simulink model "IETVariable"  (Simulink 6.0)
settings: Solver=ode45  StartTime=0.0  StopTime=10  RelTol=1e-3
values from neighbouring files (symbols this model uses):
  b = S/Sm    (= 0.1)    [Constantes.m]    (also in ConstantesBck.m)
  beta = 0.95    [Constantes.m]    (also in ConstantesBck.m; ResCourV1.m = 1; ResCrV1.m = 1; ResEnerV1.m = 1)
  C = 1    [Constantes.m]    (also in ConstantesBck.m)
  Cdl = 603E-9    (= 6.03e-07)    [Constantes.m]    (also in ConstantesBck.m; ResCourV1.m = 7.313e-07; ResCrV1.m = 7.313e-07; ResEnerV1.m = 7.313e-07)
  Cmem = 1E-6*Sm*(1-b)    (= 2.826e-08)    [Constantes.m]    (also in ConstantesBck.m = 3.14e-11; ImpedanceZtissus.m = 4e-08; Ztissus.m = 4e-08; CalculCharge.m = 1)
  Fact = 10^2    (= 100)    [Constantes.m]    (also in ConstantesBck.m)
  gk = 36    [Constantes.m]    (also in ConstantesBck.m; sim_hh.m)
  gl = 0.3    [Constantes.m]    (also in ConstantesBck.m; sim_hh.m)
  gna = 120    [Constantes.m]    (also in ConstantesBck.m; sim_hh.m)
  h0 = 0.5961    [Constantes.m]    (also in ConstantesBck.m)
  m0 = 0.0529    [Constantes.m]    (also in ConstantesBck.m)
  mK = 0    [Constantes.m]    (also in ConstantesBck.m)
  mL = 0    [Constantes.m]    (also in ConstantesBck.m)
  mNa = 0    [Constantes.m]    (also in ConstantesBck.m)
  n0 = 0.3177    [Constantes.m]    (also in ConstantesBck.m)
  rapportIE = 10    [Constantes.m]
  Rcan = 6.398E3*Sm*(1-b)    (= 180.80748)    [Constantes.m]    (also in ConstantesBck.m = 0.03454; ImpedanceZtissus.m = 44; Ztissus.m = 44)
  Rct = 185.6E3    (= 185600)    [Constantes.m]    (also in ConstantesBck.m; ResCourV1.m = 605200; ResCrV1.m = 605200; ResEnerV1.m = 605200)
  Rext = 2.9E3    (= 2900)    [Constantes.m]    (also in ConstantesBck.m)
  Rint = 2.9E2    (= 290)    [Constantes.m]    (also in ConstantesBck.m = 400)
  sigma = 66466    [Constantes.m]    (also in ConstantesBck.m; ResCourV1.m = 68000; ResCrV1.m = 68000; ResEnerV1.m = 68000)
  Sm = 3.14e-2    (= 0.0314)    [Constantes.m]    (also in ConstantesBck.m = 0.000314)
  Vk = -82    [Constantes.m]    (also in ConstantesBck.m)
  Vl = -59    [Constantes.m]    (also in ConstantesBck.m)
  Vna = 45    [Constantes.m]    (also in ConstantesBck.m)
  Vr = -70    [Constantes.m]    (also in ConstantesBck.m)
undefined symbols (not defined in the file or in its folder): ln
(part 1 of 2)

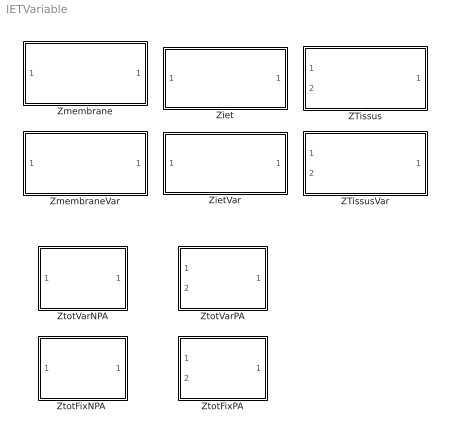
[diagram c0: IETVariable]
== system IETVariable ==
  ZTissus : Subsystem
  ZTissusVar : Subsystem
  Ziet : Subsystem
  ZietVar : Subsystem
  Zmembrane : Subsystem
  ZmembraneVar : Subsystem
  "ZtotFixNPA " : Subsystem
  ZtotFixPA : Subsystem
  ZtotVarNPA : Subsystem
  ZtotVarPA : Subsystem

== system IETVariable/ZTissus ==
  IStim : Inport  Orientation=left  Port=1  LatchInput=off
  Vref : Inport  Port=2  LatchInput=off
  Constant : Constant
  Contrôleur : Stateflow chart  Orientation=left
  Divide : Product  Inputs=*/  OutScaling=2^-10
  Divide1 : Product  Inputs=*/  OutScaling=2^-10
  Divide2 : Product  Inputs=*/  OutScaling=2^-10
  Gain2 : Gain  Gain=Rext
  Sum1 : Sum  Inputs=|++
  ZTissusInt : Subsystem
  Vout : Outport  Orientation=left
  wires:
  Constant/1 -> Divide/1, Divide1/1, Divide2/1
  ZTissusInt/1(Vout) -> Divide/2
  Gain2/1 -> Divide1/2
  Divide/1 -> Sum1/1
  Divide1/1 -> Sum1/2
  Sum1/1 -> Divide2/2
  Vref/1 -> ZTissusInt/2(VRefIn)
  Divide2/1 -> Contrôleur/2(calc)
  Contrôleur/2(temp) -> ZTissusInt/1(InStim), Gain2/1
  IStim/1 -> Contrôleur/1(u)
  Contrôleur/1(y) -> Vout/1

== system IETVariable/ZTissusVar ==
  IStim : Inport  Orientation=left  Port=1  LatchInput=off
  Vref : Inport  Port=2  LatchInput=off
  Constant : Constant
  Contrôleur : Stateflow chart  Orientation=left
  Divide : Product  Inputs=*/  OutScaling=2^-10
  Divide1 : Product  Inputs=*/  OutScaling=2^-10
  Divide2 : Product  Inputs=*/  OutScaling=2^-10
  Rext1 : Fcn  Expr=u*(1.6342*((abs(u)*1E6)^0.1267))*1E3
  Sum1 : Sum  Inputs=|++
  ZTissusInt1 : Subsystem
  Vout : Outport  Orientation=left
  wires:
  Constant/1 -> Divide/1, Divide1/1, Divide2/1
  ZTissusInt1/1(Vout) -> Divide/2
  Rext1/1 -> Divide1/2
  Divide/1 -> Sum1/1
  Divide1/1 -> Sum1/2
  Sum1/1 -> Divide2/2
  Vref/1 -> ZTissusInt1/2(VRefIn)
  Divide2/1 -> Contrôleur/2(calc)
  Contrôleur/2(temp) -> Rext1/1, ZTissusInt1/1(InStim)
  IStim/1 -> Contrôleur/1(u)
  Contrôleur/1(y) -> Vout/1

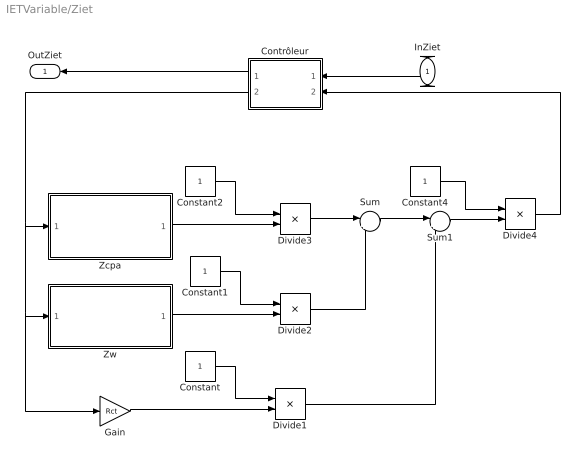
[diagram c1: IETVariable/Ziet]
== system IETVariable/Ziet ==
  InZiet : Inport  Orientation=left  Port=1  LatchInput=off
  Constant{,1..2,4} (4 alike) : Constant
  Contrôleur : Stateflow chart  Orientation=left
  Divide{1..4} (4 alike) : Product  Inputs=*/  OutScaling=2^-10
  Gain : Gain  Gain=Rct
  Sum : Sum  Inputs=|++
  Sum1 : Sum  Inputs=|++
  Zcpa : Subsystem
  Zw : Subsystem
  OutZiet : Outport  Orientation=left
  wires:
  Constant/1 -> Divide1/1
  Constant1/1 -> Divide2/1
  Constant2/1 -> Divide3/1
  Zcpa/1(OutZcpa) -> Divide3/2
  Zw/1(OutZw) -> Divide2/2
  Divide3/1 -> Sum/1
  Constant4/1 -> Divide4/1
  Divide2/1 -> Sum/2
  Sum/1 -> Sum1/1
  Divide1/1 -> Sum1/2
  Sum1/1 -> Divide4/2
  Divide4/1 -> Contrôleur/2(calc)
  Gain/1 -> Divide1/2
  InZiet/1 -> Contrôleur/1(u)
  Contrôleur/1(y) -> OutZiet/1
  Contrôleur/2(temp) -> Zcpa/1(InZcpa), Zw/1(InZw), Gain/1

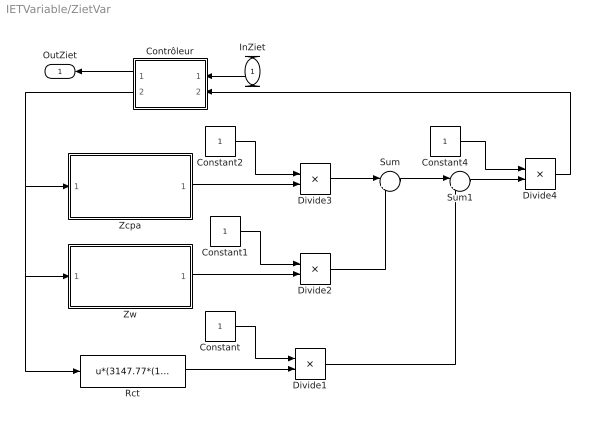
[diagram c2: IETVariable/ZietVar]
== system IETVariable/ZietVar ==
  InZiet : Inport  Orientation=left  Port=1  LatchInput=off
  Constant{,1..2,4} (4 alike) : Constant
  Contrôleur : Stateflow chart  Orientation=left
  Divide{1..4} (4 alike) : Product  Inputs=*/  OutScaling=2^-10
  Rct : Fcn  Expr=u*(3147.77*(1/((1E6*abs(u))^0.7199)))*1000
  Sum : Sum  Inputs=|++
  Sum1 : Sum  Inputs=|++
  Zcpa : Subsystem
  Zw : Subsystem
  OutZiet : Outport  Orientation=left
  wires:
  Constant/1 -> Divide1/1
  Constant1/1 -> Divide2/1
  Constant2/1 -> Divide3/1
  Zcpa/1(OutZcpa) -> Divide3/2
  Zw/1(OutZw) -> Divide2/2
  Rct/1 -> Divide1/2
  Divide3/1 -> Sum/1
  Constant4/1 -> Divide4/1
  Divide2/1 -> Sum/2
  Sum/1 -> Sum1/1
  Divide1/1 -> Sum1/2
  Sum1/1 -> Divide4/2
  Contrôleur/2(temp) -> Rct/1, Zw/1(InZw), Zcpa/1(InZcpa)
  InZiet/1 -> Contrôleur/1(u)
  Contrôleur/1(y) -> OutZiet/1
  Divide4/1 -> Contrôleur/2(calc)

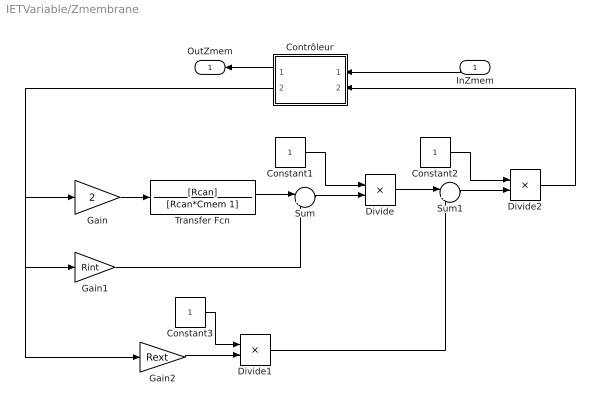
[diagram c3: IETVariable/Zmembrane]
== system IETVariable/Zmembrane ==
  InZmem : Inport  Orientation=left  Port=1  LatchInput=off
  Constant1 : Constant
  Constant2 : Constant
  Constant3 : Constant
  Contrôleur : Stateflow chart  Orientation=left
  Divide : Product  Inputs=*/  OutScaling=2^-10
  Divide1 : Product  Inputs=*/  OutScaling=2^-10
  Divide2 : Product  Inputs=*/  OutScaling=2^-10
  Gain : Gain  Gain=2
  Gain1 : Gain  Gain=Rint
  Gain2 : Gain  Gain=Rext
  Sum : Sum  Inputs=|++
  Sum1 : Sum  Inputs=|++
  Transfer Fcn : TransferFcn  Numerator=[Rcan]  Denominator=[Rcan*Cmem 1]
  OutZmem : Outport  Orientation=left
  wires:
  Gain/1 -> Transfer Fcn/1
  Transfer Fcn/1 -> Sum/1
  Sum/1 -> Divide/2
  Gain2/1 -> Divide1/2
  Constant1/1 -> Divide/1
  Divide/1 -> Sum1/1
  Constant2/1 -> Divide2/1
  Sum1/1 -> Divide2/2
  Gain1/1 -> Sum/2
  Divide1/1 -> Sum1/2
  Divide2/1 -> Contrôleur/2(calc)
  Constant3/1 -> Divide1/1
  Contrôleur/2(temp) -> Gain2/1, Gain1/1, Gain/1
  InZmem/1 -> Contrôleur/1(u)
  Contrôleur/1(y) -> OutZmem/1

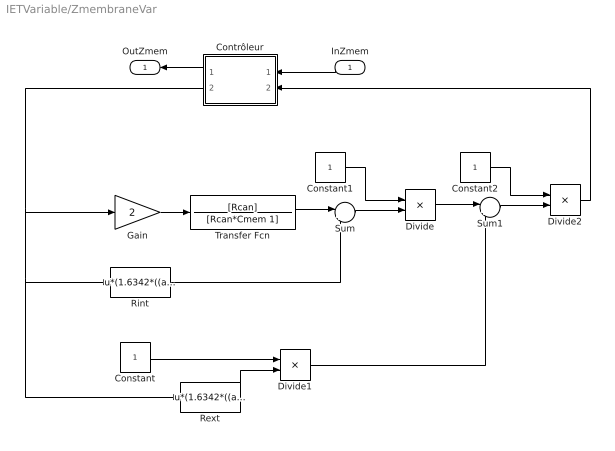
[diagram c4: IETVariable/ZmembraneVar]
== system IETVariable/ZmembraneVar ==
  InZmem : Inport  Orientation=left  Port=1  LatchInput=off
  Constant : Constant
  Constant1 : Constant
  Constant2 : Constant
  Contrôleur : Stateflow chart  Orientation=left
  Divide : Product  Inputs=*/  OutScaling=2^-10
  Divide1 : Product  Inputs=*/  OutScaling=2^-10
  Divide2 : Product  Inputs=*/  OutScaling=2^-10
  Gain : Gain  Gain=2
  Rext : Fcn  Expr=u*(1.6342*((abs(u)*1E6)^0.1267))*1E3
  Rint : Fcn  Expr=u*(1.6342*((abs(u)*1E6)^0.1267))*1E3/rapportIE
  Sum : Sum  Inputs=|++
  Sum1 : Sum  Inputs=|++
  Transfer Fcn : TransferFcn  Numerator=[Rcan]  Denominator=[Rcan*Cmem 1]
  OutZmem : Outport  Orientation=left
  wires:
  Gain/1 -> Transfer Fcn/1
  Transfer Fcn/1 -> Sum/1
  Sum/1 -> Divide/2
  Rext/1 -> Divide1/2
  Constant1/1 -> Divide/1
  Constant/1 -> Divide1/1
  Divide/1 -> Sum1/1
  Constant2/1 -> Divide2/1
  Sum1/1 -> Divide2/2
  Rint/1 -> Sum/2
  Divide1/1 -> Sum1/2
  Contrôleur/2(temp) -> Rext/1, Rint/1, Gain/1
  Divide2/1 -> Contrôleur/2(calc)
  InZmem/1 -> Contrôleur/1(u)
  Contrôleur/1(y) -> OutZmem/1

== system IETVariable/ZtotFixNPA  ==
  InZtot : Inport  Port=1  LatchInput=off
  Gain : Gain
  Sum : Sum  Inputs=|++
  Ziet : Subsystem
  Zmembrane : Subsystem
  OutZtot : Outport
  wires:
  Ziet/1(OutZiet) -> Gain/1
  Zmembrane/1(OutZmem) -> Sum/1
  InZtot/1 -> Zmembrane/1(InZmem), Ziet/1(InZiet)
  Gain/1 -> Sum/2
  Sum/1 -> OutZtot/1

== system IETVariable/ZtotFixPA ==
  InZtot : Inport  Port=1  LatchInput=off
  InVref : Inport  Port=2  LatchInput=off
  Gain : Gain
  Sum : Sum  Inputs=|++
  ZTissus : Subsystem
  Ziet : Subsystem
  OutZtot : Outport
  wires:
  ZTissus/1(Vout) -> Sum/2
  Ziet/1(OutZiet) -> Gain/1
  InZtot/1 -> Ziet/1(InZiet), ZTissus/1(IStim)
  Sum/1 -> OutZtot/1
  Gain/1 -> Sum/1
  InVref/1 -> ZTissus/2(Vref)

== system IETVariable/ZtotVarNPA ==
  InZtot : Inport  Port=1  LatchInput=off
  Gain : Gain
  Sum : Sum  Inputs=|++
  ZietVar : Subsystem
  ZmembraneVar : Subsystem
  OutZtot : Outport
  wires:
  ZietVar/1(OutZiet) -> Gain/1
  ZmembraneVar/1(OutZmem) -> Sum/1
  InZtot/1 -> ZmembraneVar/1(InZmem), ZietVar/1(InZiet)
  Gain/1 -> Sum/2
  Sum/1 -> OutZtot/1

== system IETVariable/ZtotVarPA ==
  InZtot : Inport  Port=1  LatchInput=off
  InVref : Inport  Port=2  LatchInput=off
  Gain : Gain
  Sum : Sum  Inputs=|++
  ZTissusVar : Subsystem
  ZietVar : Subsystem
  OutZtot : Outport
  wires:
  ZietVar/1(OutZiet) -> Gain/1
  ZTissusVar/1(Vout) -> Sum/1
  InZtot/1 -> ZietVar/1(InZiet), ZTissusVar/1(IStim)
  Gain/1 -> Sum/2
  Sum/1 -> OutZtot/1
  InVref/1 -> ZTissusVar/2(Vref)

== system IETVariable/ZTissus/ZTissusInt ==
  InStim : Inport  Orientation=down  Port=1  LatchInput=off
  VRefIn : Inport  Port=2  LatchInput=off
  Gain1 : Gain  Gain=Rint
  Gain2 : Gain  Gain=-1
  Gain3 : Gain
  Gain4 : Gain  Gain=-1
  Modele HH : Subsystem
  Modele HHRetour : Subsystem
  Sum1 : Sum  Inputs=|+++
  Sum2 : Sum  Inputs=|+-
  Vout : Outport
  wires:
  Modele HH/1(HHout) -> Gain3/1
  Modele HHRetour/1(HHout) -> Gain4/1
  Gain1/1 -> Sum1/2
  InStim/1 -> Gain1/1, Modele HHRetour/1(HHin), Gain2/1
  Sum2/1 -> Modele HH/2(VRefIn)
  Sum1/1 -> Vout/1, Sum2/2
  VRefIn/1 -> Modele HHRetour/2(VRefIn), Sum2/1
  Gain3/1 -> Sum1/1
  Gain4/1 -> Sum1/3
  Gain2/1 -> Modele HH/1(HHin)

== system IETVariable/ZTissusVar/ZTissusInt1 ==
  InStim : Inport  Orientation=down  Port=1  LatchInput=off
  VRefIn : Inport  Port=2  LatchInput=off
  Gain2 : Gain  Gain=-1
  Gain3 : Gain
  Gain4 : Gain  Gain=-1
  Modele HH : Subsystem
  Modele HHRetour : Subsystem
  Rint : Fcn  Expr=u*(1.6342*((abs(u)*1E6)^0.1267))*1E3/rapportIE
  "Scope2 " : Scope
  Scope3 : Scope
  Sum1 : Sum  Inputs=|+++
  Sum2 : Sum  Inputs=|+-
  Vout : Outport
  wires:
  Modele HH/1(HHout) -> Gain3/1
  Modele HHRetour/1(HHout) -> Gain4/1
  Rint/1 -> Sum1/2
  InStim/1 -> Modele HHRetour/1(HHin), Rint/1, Gain2/1
  Sum2/1 -> Modele HH/2(VRefIn)
  Sum1/1 -> Vout/1, Sum2/2
  VRefIn/1 -> Modele HHRetour/2(VRefIn), Sum2/1
  Gain3/1 -> Sum1/1, "Scope2 "/1
  Gain4/1 -> Sum1/3, Scope3/1
  Gain2/1 -> Modele HH/1(HHin)

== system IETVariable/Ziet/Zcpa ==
  InZcpa : Inport  Port=1  LatchInput=off
  Fcn : Fcn  Expr=u(1)^beta
  Transfer Fcn : TransferFcn  Denominator=[Cdl 0]
  OutZcpa : Outport
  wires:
  Transfer Fcn/1 -> Fcn/1
  InZcpa/1 -> Transfer Fcn/1
  Fcn/1 -> OutZcpa/1

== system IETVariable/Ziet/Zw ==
  InZw : Inport  Port=1  LatchInput=off
  Gain : Gain  Gain=sigma
  Math Function : Math  Operator=sqrt
  Transfer Fcn : TransferFcn  Numerator=[2]  Denominator=[1 0]
  OutZw : Outport
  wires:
  Transfer Fcn/1 -> Math Function/1
  Math Function/1 -> Gain/1
  Gain/1 -> OutZw/1
  InZw/1 -> Transfer Fcn/1

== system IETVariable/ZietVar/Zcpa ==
  InZcpa : Inport  Port=1  LatchInput=off
  Cdl : Fcn  Expr=u*1E9/(918.15-80.854*ln(abs(u)*1E6))
  Fcn : Fcn  Expr=u(1)^beta
  Transfer Fcn : TransferFcn  Denominator=[1 0]
  OutZcpa : Outport
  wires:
  Transfer Fcn/1 -> Fcn/1
  InZcpa/1 -> Cdl/1
  Fcn/1 -> OutZcpa/1
  Cdl/1 -> Transfer Fcn/1

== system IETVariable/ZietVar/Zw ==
  InZw : Inport  Port=1  LatchInput=off
  Math Function : Math  Operator=sqrt
  Product : Product
  Transfer Fcn : TransferFcn  Numerator=[2]  Denominator=[1 0]
  sigma : Fcn  Expr=(67202-0.0688*((1E6*abs(u))^2)-11.273*(1E6*abs(u)))
  OutZw : Outport
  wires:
  Transfer Fcn/1 -> Math Function/1
  InZw/1 -> Transfer Fcn/1, sigma/1
  Math Function/1 -> Product/1
  sigma/1 -> Product/2
  Product/1 -> OutZw/1

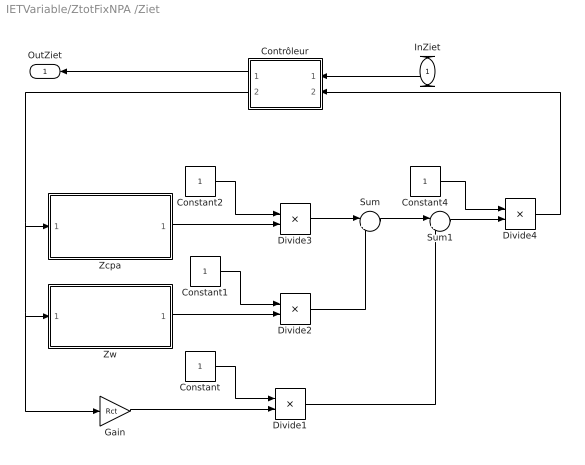
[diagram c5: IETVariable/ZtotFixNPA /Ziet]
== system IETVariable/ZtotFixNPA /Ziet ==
  InZiet : Inport  Orientation=left  Port=1  LatchInput=off
  Constant{,1..2,4} (4 alike) : Constant
  Contrôleur : Stateflow chart  Orientation=left
  Divide{1..4} (4 alike) : Product  Inputs=*/  OutScaling=2^-10
  Gain : Gain  Gain=Rct
  Sum : Sum  Inputs=|++
  Sum1 : Sum  Inputs=|++
  Zcpa : Subsystem
  Zw : Subsystem
  OutZiet : Outport  Orientation=left
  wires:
  Constant/1 -> Divide1/1
  Constant1/1 -> Divide2/1
  Constant2/1 -> Divide3/1
  Zcpa/1(OutZcpa) -> Divide3/2
  Zw/1(OutZw) -> Divide2/2
  Divide3/1 -> Sum/1
  Constant4/1 -> Divide4/1
  Divide2/1 -> Sum/2
  Sum/1 -> Sum1/1
  Divide1/1 -> Sum1/2
  Sum1/1 -> Divide4/2
  Divide4/1 -> Contrôleur/2(calc)
  Gain/1 -> Divide1/2
  InZiet/1 -> Contrôleur/1(u)
  Contrôleur/1(y) -> OutZiet/1
  Contrôleur/2(temp) -> Zcpa/1(InZcpa), Zw/1(InZw), Gain/1

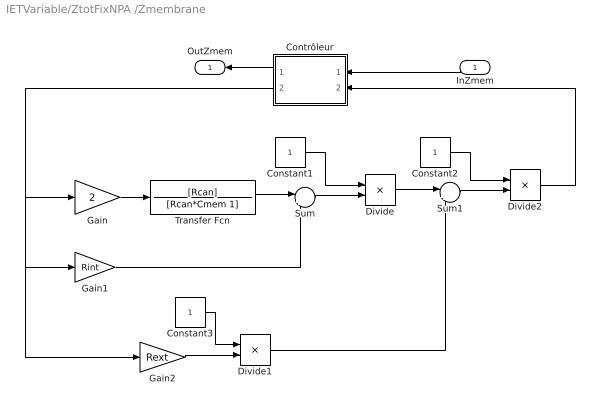
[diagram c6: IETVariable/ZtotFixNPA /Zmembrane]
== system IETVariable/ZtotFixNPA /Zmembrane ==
  InZmem : Inport  Orientation=left  Port=1  LatchInput=off
  Constant1 : Constant
  Constant2 : Constant
  Constant3 : Constant
  Contrôleur : Stateflow chart  Orientation=left
  Divide : Product  Inputs=*/  OutScaling=2^-10
  Divide1 : Product  Inputs=*/  OutScaling=2^-10
  Divide2 : Product  Inputs=*/  OutScaling=2^-10
  Gain : Gain  Gain=2
  Gain1 : Gain  Gain=Rint
  Gain2 : Gain  Gain=Rext
  Sum : Sum  Inputs=|++
  Sum1 : Sum  Inputs=|++
  Transfer Fcn : TransferFcn  Numerator=[Rcan]  Denominator=[Rcan*Cmem 1]
  OutZmem : Outport  Orientation=left
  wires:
  Gain/1 -> Transfer Fcn/1
  Transfer Fcn/1 -> Sum/1
  Sum/1 -> Divide/2
  Gain2/1 -> Divide1/2
  Constant1/1 -> Divide/1
  Divide/1 -> Sum1/1
  Constant2/1 -> Divide2/1
  Sum1/1 -> Divide2/2
  Gain1/1 -> Sum/2
  Divide1/1 -> Sum1/2
  Divide2/1 -> Contrôleur/2(calc)
  Constant3/1 -> Divide1/1
  Contrôleur/2(temp) -> Gain2/1, Gain1/1, Gain/1
  InZmem/1 -> Contrôleur/1(u)
  Contrôleur/1(y) -> OutZmem/1

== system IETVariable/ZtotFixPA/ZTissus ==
  IStim : Inport  Orientation=left  Port=1  LatchInput=off
  Vref : Inport  Port=2  LatchInput=off
  Constant : Constant
  Contrôleur : Stateflow chart  Orientation=left
  Divide : Product  Inputs=*/  OutScaling=2^-10
  Divide1 : Product  Inputs=*/  OutScaling=2^-10
  Divide2 : Product  Inputs=*/  OutScaling=2^-10
  Gain2 : Gain  Gain=Rext
  Sum1 : Sum  Inputs=|++
  ZTissusInt : Subsystem
  Vout : Outport  Orientation=left
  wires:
  Constant/1 -> Divide/1, Divide1/1, Divide2/1
  ZTissusInt/1(Vout) -> Divide/2
  Gain2/1 -> Divide1/2
  Divide/1 -> Sum1/1
  Divide1/1 -> Sum1/2
  Sum1/1 -> Divide2/2
  Vref/1 -> ZTissusInt/2(VRefIn)
  Divide2/1 -> Contrôleur/2(calc)
  Contrôleur/2(temp) -> ZTissusInt/1(InStim), Gain2/1
  IStim/1 -> Contrôleur/1(u)
  Contrôleur/1(y) -> Vout/1

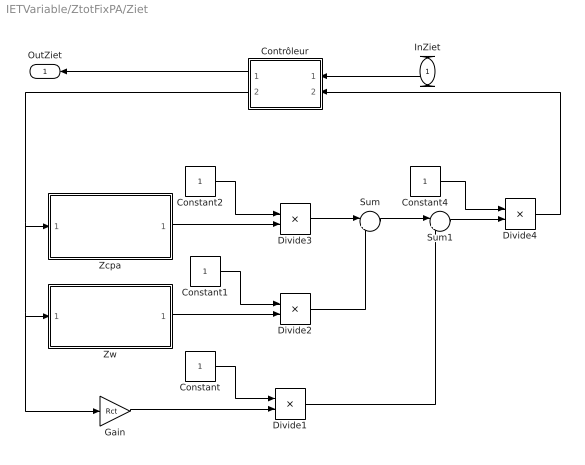
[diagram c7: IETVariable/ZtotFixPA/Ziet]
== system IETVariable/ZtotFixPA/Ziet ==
  InZiet : Inport  Orientation=left  Port=1  LatchInput=off
  Constant{,1..2,4} (4 alike) : Constant
  Contrôleur : Stateflow chart  Orientation=left
  Divide{1..4} (4 alike) : Product  Inputs=*/  OutScaling=2^-10
  Gain : Gain  Gain=Rct
  Sum : Sum  Inputs=|++
  Sum1 : Sum  Inputs=|++
  Zcpa : Subsystem
  Zw : Subsystem
  OutZiet : Outport  Orientation=left
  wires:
  Constant/1 -> Divide1/1
  Constant1/1 -> Divide2/1
  Constant2/1 -> Divide3/1
  Zcpa/1(OutZcpa) -> Divide3/2
  Zw/1(OutZw) -> Divide2/2
  Divide3/1 -> Sum/1
  Constant4/1 -> Divide4/1
  Divide2/1 -> Sum/2
  Sum/1 -> Sum1/1
  Divide1/1 -> Sum1/2
  Sum1/1 -> Divide4/2
  Divide4/1 -> Contrôleur/2(calc)
  Gain/1 -> Divide1/2
  InZiet/1 -> Contrôleur/1(u)
  Contrôleur/1(y) -> OutZiet/1
  Contrôleur/2(temp) -> Zcpa/1(InZcpa), Zw/1(InZw), Gain/1

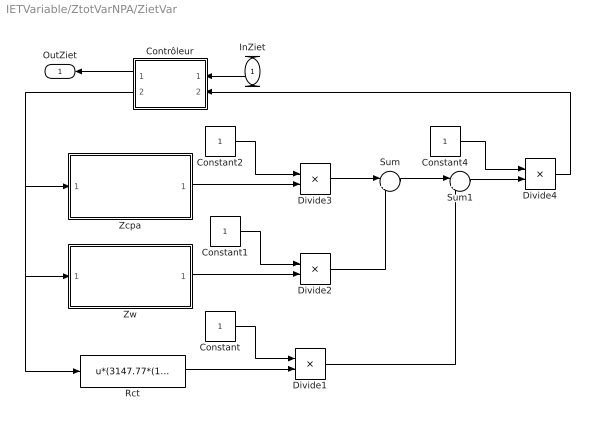
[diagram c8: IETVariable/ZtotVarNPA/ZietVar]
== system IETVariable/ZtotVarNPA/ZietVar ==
  InZiet : Inport  Orientation=left  Port=1  LatchInput=off
  Constant{,1..2,4} (4 alike) : Constant
  Contrôleur : Stateflow chart  Orientation=left
  Divide{1..4} (4 alike) : Product  Inputs=*/  OutScaling=2^-10
  Rct : Fcn  Expr=u*(3147.77*(1/((1E6*abs(u))^0.7199)))*1000
  Sum : Sum  Inputs=|++
  Sum1 : Sum  Inputs=|++
  Zcpa : Subsystem
  Zw : Subsystem
  OutZiet : Outport  Orientation=left
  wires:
  Constant/1 -> Divide1/1
  Constant1/1 -> Divide2/1
  Constant2/1 -> Divide3/1
  Zcpa/1(OutZcpa) -> Divide3/2
  Zw/1(OutZw) -> Divide2/2
  Rct/1 -> Divide1/2
  Divide3/1 -> Sum/1
  Constant4/1 -> Divide4/1
  Divide2/1 -> Sum/2
  Sum/1 -> Sum1/1
  Divide1/1 -> Sum1/2
  Sum1/1 -> Divide4/2
  Contrôleur/2(temp) -> Rct/1, Zw/1(InZw), Zcpa/1(InZcpa)
  InZiet/1 -> Contrôleur/1(u)
  Contrôleur/1(y) -> OutZiet/1
  Divide4/1 -> Contrôleur/2(calc)

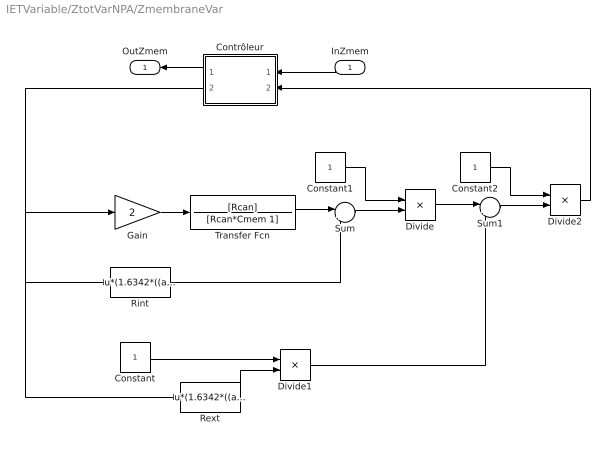
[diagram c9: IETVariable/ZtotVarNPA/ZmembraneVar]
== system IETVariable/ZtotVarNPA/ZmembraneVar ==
  InZmem : Inport  Orientation=left  Port=1  LatchInput=off
  Constant : Constant
  Constant1 : Constant
  Constant2 : Constant
  Contrôleur : Stateflow chart  Orientation=left
  Divide : Product  Inputs=*/  OutScaling=2^-10
  Divide1 : Product  Inputs=*/  OutScaling=2^-10
  Divide2 : Product  Inputs=*/  OutScaling=2^-10
  Gain : Gain  Gain=2
  Rext : Fcn  Expr=u*(1.6342*((abs(u)*1E6)^0.1267))*1E3
  Rint : Fcn  Expr=u*(1.6342*((abs(u)*1E6)^0.1267))*1E3/rapportIE
  Sum : Sum  Inputs=|++
  Sum1 : Sum  Inputs=|++
  Transfer Fcn : TransferFcn  Numerator=[Rcan]  Denominator=[Rcan*Cmem 1]
  OutZmem : Outport  Orientation=left
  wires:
  Gain/1 -> Transfer Fcn/1
  Transfer Fcn/1 -> Sum/1
  Sum/1 -> Divide/2
  Rext/1 -> Divide1/2
  Constant1/1 -> Divide/1
  Constant/1 -> Divide1/1
  Divide/1 -> Sum1/1
  Constant2/1 -> Divide2/1
  Sum1/1 -> Divide2/2
  Rint/1 -> Sum/2
  Divide1/1 -> Sum1/2
  Contrôleur/2(temp) -> Rext/1, Rint/1, Gain/1
  Divide2/1 -> Contrôleur/2(calc)
  InZmem/1 -> Contrôleur/1(u)
  Contrôleur/1(y) -> OutZmem/1

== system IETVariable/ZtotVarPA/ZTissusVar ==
  IStim : Inport  Orientation=left  Port=1  LatchInput=off
  Vref : Inport  Port=2  LatchInput=off
  Constant : Constant
  Contrôleur : Stateflow chart  Orientation=left
  Divide : Product  Inputs=*/  OutScaling=2^-10
  Divide1 : Product  Inputs=*/  OutScaling=2^-10
  Divide2 : Product  Inputs=*/  OutScaling=2^-10
  Rext1 : Fcn  Expr=u*(1.6342*((abs(u)*1E6)^0.1267))*1E3
  Sum1 : Sum  Inputs=|++
  ZTissusInt1 : Subsystem
  Vout : Outport  Orientation=left
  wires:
  Constant/1 -> Divide/1, Divide1/1, Divide2/1
  ZTissusInt1/1(Vout) -> Divide/2
  Rext1/1 -> Divide1/2
  Divide/1 -> Sum1/1
  Divide1/1 -> Sum1/2
  Sum1/1 -> Divide2/2
  Vref/1 -> ZTissusInt1/2(VRefIn)
  Divide2/1 -> Contrôleur/2(calc)
  Contrôleur/2(temp) -> Rext1/1, ZTissusInt1/1(InStim)
  IStim/1 -> Contrôleur/1(u)
  Contrôleur/1(y) -> Vout/1

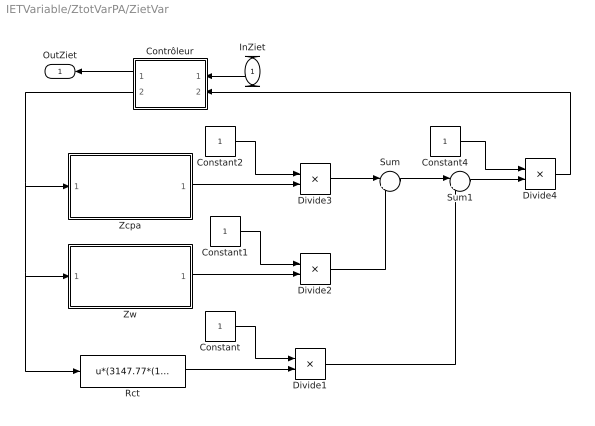
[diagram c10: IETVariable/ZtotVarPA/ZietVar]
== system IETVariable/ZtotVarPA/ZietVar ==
  InZiet : Inport  Orientation=left  Port=1  LatchInput=off
  Constant{,1..2,4} (4 alike) : Constant
  Contrôleur : Stateflow chart  Orientation=left
  Divide{1..4} (4 alike) : Product  Inputs=*/  OutScaling=2^-10
  Rct : Fcn  Expr=u*(3147.77*(1/((1E6*abs(u))^0.7199)))*1000
  Sum : Sum  Inputs=|++
  Sum1 : Sum  Inputs=|++
  Zcpa : Subsystem
  Zw : Subsystem
  OutZiet : Outport  Orientation=left
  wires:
  Constant/1 -> Divide1/1
  Constant1/1 -> Divide2/1
  Constant2/1 -> Divide3/1
  Zcpa/1(OutZcpa) -> Divide3/2
  Zw/1(OutZw) -> Divide2/2
  Rct/1 -> Divide1/2
  Divide3/1 -> Sum/1
  Constant4/1 -> Divide4/1
  Divide2/1 -> Sum/2
  Sum/1 -> Sum1/1
  Divide1/1 -> Sum1/2
  Sum1/1 -> Divide4/2
  Contrôleur/2(temp) -> Rct/1, Zw/1(InZw), Zcpa/1(InZcpa)
  InZiet/1 -> Contrôleur/1(u)
  Contrôleur/1(y) -> OutZiet/1
  Divide4/1 -> Contrôleur/2(calc)

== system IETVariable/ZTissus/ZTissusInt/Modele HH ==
  HHin : Inport  Port=1  LatchInput=off
  VRefIn : Inport  Port=2  LatchInput=off
  FK : Subsystem
  FL : Fcn  Expr=gl*(u-Vl)
  FNa : Subsystem
  Gain : Gain  Gain=(1-b)/C
  Gain1 : Gain  Gain=1/(Sm*(1-b))
  Gain2 : Gain  Gain=1+mK*(b/(1-b))
  Gain3 : Gain  Gain=1+mL*(b/(1-b))
  Gain4 : Gain  Gain=1+mNa*(b/(1-b))
  Integrator : Integrator  InitialCondition=Vr
  Sum : Sum  Inputs=|---+
  Sum1 : Sum  Inputs=|++
  HHout : Outport
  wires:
  Sum/1 -> Gain/1
  Gain/1 -> Integrator/1
  FK/1(FKout) -> Gain4/1
  FNa/1(FNaOut) -> Gain2/1
  FL/1 -> Gain3/1
  HHin/1 -> Gain1/1
  Integrator/1 -> Sum1/1
  Sum1/1 -> HHout/1, FNa/1(FNaIn), FL/1, FK/1(FKIn)
  VRefIn/1 -> Sum1/2
  Gain1/1 -> Sum/4
  Gain4/1 -> Sum/1
  Gain2/1 -> Sum/2
  Gain3/1 -> Sum/3

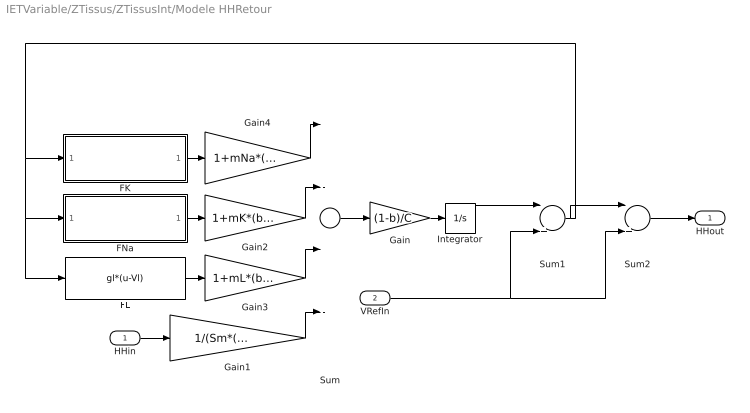
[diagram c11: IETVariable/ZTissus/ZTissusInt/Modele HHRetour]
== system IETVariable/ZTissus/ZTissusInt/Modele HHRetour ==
  HHin : Inport  Port=1  LatchInput=off
  VRefIn : Inport  Port=2  LatchInput=off
  FK : Subsystem
  FL : Fcn  Expr=gl*(u-Vl)
  FNa : Subsystem
  Gain : Gain  Gain=(1-b)/C
  Gain1 : Gain  Gain=1/(Sm*(1-b)*Fact)
  Gain2 : Gain  Gain=1+mK*(b/(1-b))
  Gain3 : Gain  Gain=1+mL*(b/(1-b))
  Gain4 : Gain  Gain=1+mNa*(b/(1-b))
  Integrator : Integrator  InitialCondition=Vr
  Sum : Sum  Inputs=|---+
  Sum1 : Sum  Inputs=|++
  Sum2 : Sum  Inputs=|+-
  HHout : Outport
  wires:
  Sum/1 -> Gain/1
  Gain/1 -> Integrator/1
  FK/1(FKout) -> Gain4/1
  FNa/1(FNaOut) -> Gain2/1
  FL/1 -> Gain3/1
  HHin/1 -> Gain1/1
  Integrator/1 -> Sum1/1
  Sum1/1 -> FNa/1(FNaIn), FL/1, FK/1(FKIn), Sum2/1
  VRefIn/1 -> Sum1/2, Sum2/2
  Gain1/1 -> Sum/4
  Gain4/1 -> Sum/1
  Gain2/1 -> Sum/2
  Gain3/1 -> Sum/3
  Sum2/1 -> HHout/1

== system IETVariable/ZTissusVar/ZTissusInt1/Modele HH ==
  HHin : Inport  Port=1  LatchInput=off
  VRefIn : Inport  Port=2  LatchInput=off
  FK : Subsystem
  FL : Fcn  Expr=gl*(u-Vl)
  FNa : Subsystem
  Gain : Gain  Gain=(1-b)/C
  Gain1 : Gain  Gain=1/(Sm*(1-b))
  Gain2 : Gain  Gain=1+mK*(b/(1-b))
  Gain3 : Gain  Gain=1+mL*(b/(1-b))
  Gain4 : Gain  Gain=1+mNa*(b/(1-b))
  Integrator : Integrator  InitialCondition=Vr
  Sum : Sum  Inputs=|---+
  Sum1 : Sum  Inputs=|++
  HHout : Outport
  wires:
  Sum/1 -> Gain/1
  Gain/1 -> Integrator/1
  FK/1(FKout) -> Gain4/1
  FNa/1(FNaOut) -> Gain2/1
  FL/1 -> Gain3/1
  HHin/1 -> Gain1/1
  Integrator/1 -> Sum1/1
  Sum1/1 -> HHout/1, FNa/1(FNaIn), FL/1, FK/1(FKIn)
  VRefIn/1 -> Sum1/2
  Gain1/1 -> Sum/4
  Gain4/1 -> Sum/1
  Gain2/1 -> Sum/2
  Gain3/1 -> Sum/3

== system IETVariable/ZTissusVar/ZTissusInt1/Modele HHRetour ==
  HHin : Inport  Port=1  LatchInput=off
  VRefIn : Inport  Port=2  LatchInput=off
  FK : Subsystem
  FL : Fcn  Expr=gl*(u-Vl)
  FNa : Subsystem
  Gain : Gain  Gain=(1-b)/C
  Gain1 : Gain  Gain=1/(Sm*(1-b)*Fact)
  Gain2 : Gain  Gain=1+mK*(b/(1-b))
  Gain3 : Gain  Gain=1+mL*(b/(1-b))
  Gain4 : Gain  Gain=1+mNa*(b/(1-b))
  Integrator : Integrator  InitialCondition=Vr
  Sum : Sum  Inputs=|---+
  Sum1 : Sum  Inputs=|++
  Sum2 : Sum  Inputs=|+-
  HHout : Outport
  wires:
  Sum/1 -> Gain/1
  Gain/1 -> Integrator/1
  FK/1(FKout) -> Gain4/1
  FNa/1(FNaOut) -> Gain2/1
  FL/1 -> Gain3/1
  HHin/1 -> Gain1/1
  Integrator/1 -> Sum1/1
  Sum1/1 -> FNa/1(FNaIn), FL/1, FK/1(FKIn), Sum2/1
  VRefIn/1 -> Sum1/2, Sum2/2
  Gain1/1 -> Sum/4
  Gain4/1 -> Sum/1
  Gain2/1 -> Sum/2
  Gain3/1 -> Sum/3
  Sum2/1 -> HHout/1

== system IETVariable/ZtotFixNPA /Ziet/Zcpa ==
  InZcpa : Inport  Port=1  LatchInput=off
  Fcn : Fcn  Expr=u^beta
  Transfer Fcn : TransferFcn  Denominator=[Cdl 0]
  OutZcpa : Outport
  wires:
  Transfer Fcn/1 -> Fcn/1
  InZcpa/1 -> Transfer Fcn/1
  Fcn/1 -> OutZcpa/1

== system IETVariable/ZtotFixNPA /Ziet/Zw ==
  InZw : Inport  Port=1  LatchInput=off
  Gain : Gain  Gain=sigma
  Math Function : Math  Operator=sqrt
  Transfer Fcn : TransferFcn  Numerator=[2]  Denominator=[1 0]
  OutZw : Outport
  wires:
  Transfer Fcn/1 -> Math Function/1
  Math Function/1 -> Gain/1
  Gain/1 -> OutZw/1
  InZw/1 -> Transfer Fcn/1

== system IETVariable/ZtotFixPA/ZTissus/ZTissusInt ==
  InStim : Inport  Orientation=down  Port=1  LatchInput=off
  VRefIn : Inport  Port=2  LatchInput=off
  Gain1 : Gain  Gain=Rint
  Gain2 : Gain  Gain=-1
  Gain3 : Gain
  Gain4 : Gain  Gain=-1
  Modele HH : Subsystem
  Modele HHRetour : Subsystem
  Sum1 : Sum  Inputs=|+++
  Sum2 : Sum  Inputs=|+-
  Vout : Outport
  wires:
  Modele HH/1(HHout) -> Gain3/1
  Modele HHRetour/1(HHout) -> Gain4/1
  Gain1/1 -> Sum1/2
  InStim/1 -> Gain1/1, Modele HHRetour/1(HHin), Gain2/1
  Sum2/1 -> Modele HH/2(VRefIn)
  Sum1/1 -> Vout/1, Sum2/2
  VRefIn/1 -> Modele HHRetour/2(VRefIn), Sum2/1
  Gain3/1 -> Sum1/1
  Gain4/1 -> Sum1/3
  Gain2/1 -> Modele HH/1(HHin)

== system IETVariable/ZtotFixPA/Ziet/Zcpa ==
  InZcpa : Inport  Port=1  LatchInput=off
  Fcn : Fcn  Expr=u^beta
  Transfer Fcn : TransferFcn  Denominator=[Cdl 0]
  OutZcpa : Outport
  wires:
  Transfer Fcn/1 -> Fcn/1
  InZcpa/1 -> Transfer Fcn/1
  Fcn/1 -> OutZcpa/1

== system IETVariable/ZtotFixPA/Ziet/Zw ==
  InZw : Inport  Port=1  LatchInput=off
  Gain : Gain  Gain=sigma
  Math Function : Math  Operator=sqrt
  Transfer Fcn : TransferFcn  Numerator=[2]  Denominator=[1 0]
  OutZw : Outport
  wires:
  Transfer Fcn/1 -> Math Function/1
  Math Function/1 -> Gain/1
  Gain/1 -> OutZw/1
  InZw/1 -> Transfer Fcn/1

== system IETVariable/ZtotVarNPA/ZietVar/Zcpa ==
  InZcpa : Inport  Port=1  LatchInput=off
  Cdl : Fcn  Expr=u*1E9/(918.15-80.854*ln(abs(u)*1E6))
  Fcn : Fcn  Expr=u^beta
  Transfer Fcn : TransferFcn  Denominator=[1 0]
  OutZcpa : Outport
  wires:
  Transfer Fcn/1 -> Fcn/1
  InZcpa/1 -> Cdl/1
  Fcn/1 -> OutZcpa/1
  Cdl/1 -> Transfer Fcn/1

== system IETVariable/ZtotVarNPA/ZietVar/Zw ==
  InZw : Inport  Port=1  LatchInput=off
  Math Function : Math  Operator=sqrt
  Product : Product
  Transfer Fcn : TransferFcn  Numerator=[2]  Denominator=[1 0]
  sigma : Fcn  Expr=(67202-0.0688*((1E6*abs(u))^2)-11.273*(1E6*abs(u)))
  OutZw : Outport
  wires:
  Transfer Fcn/1 -> Math Function/1
  InZw/1 -> Transfer Fcn/1, sigma/1
  Math Function/1 -> Product/1
  sigma/1 -> Product/2
  Product/1 -> OutZw/1

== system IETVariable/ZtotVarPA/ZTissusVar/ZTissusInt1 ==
  InStim : Inport  Orientation=down  Port=1  LatchInput=off
  VRefIn : Inport  Port=2  LatchInput=off
  Gain2 : Gain  Gain=-1
  Gain3 : Gain
  Gain4 : Gain  Gain=-1
  Modele HH : Subsystem
  Modele HHRetour : Subsystem
  Rint : Fcn  Expr=u*(1.6342*((abs(u)*1E6)^0.1267))*1E3/rapportIE
  "Scope2 " : Scope
  Scope3 : Scope
  Sum1 : Sum  Inputs=|+++
  Sum2 : Sum  Inputs=|+-
  Vout : Outport
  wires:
  Modele HH/1(HHout) -> Gain3/1
  Modele HHRetour/1(HHout) -> Gain4/1
  Rint/1 -> Sum1/2
  InStim/1 -> Modele HHRetour/1(HHin), Rint/1, Gain2/1
  Sum2/1 -> Modele HH/2(VRefIn)
  Sum1/1 -> Vout/1, Sum2/2
  VRefIn/1 -> Modele HHRetour/2(VRefIn), Sum2/1
  Gain3/1 -> Sum1/1, "Scope2 "/1
  Gain4/1 -> Sum1/3, Scope3/1
  Gain2/1 -> Modele HH/1(HHin)

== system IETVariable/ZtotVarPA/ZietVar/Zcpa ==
  InZcpa : Inport  Port=1  LatchInput=off
  Cdl : Fcn  Expr=u*1E9/(918.15-80.854*ln(abs(u)*1E6))
  Fcn : Fcn  Expr=u^beta
  Transfer Fcn : TransferFcn  Denominator=[1 0]
  OutZcpa : Outport
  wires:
  Transfer Fcn/1 -> Fcn/1
  InZcpa/1 -> Cdl/1
  Fcn/1 -> OutZcpa/1
  Cdl/1 -> Transfer Fcn/1

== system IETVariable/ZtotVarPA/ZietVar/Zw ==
  InZw : Inport  Port=1  LatchInput=off
  Math Function : Math  Operator=sqrt
  Product : Product
  Transfer Fcn : TransferFcn  Numerator=[2]  Denominator=[1 0]
  sigma : Fcn  Expr=(67202-0.0688*((1E6*abs(u))^2)-11.273*(1E6*abs(u)))
  OutZw : Outport
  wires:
  Transfer Fcn/1 -> Math Function/1
  InZw/1 -> Transfer Fcn/1, sigma/1
  Math Function/1 -> Product/1
  sigma/1 -> Product/2
  Product/1 -> OutZw/1

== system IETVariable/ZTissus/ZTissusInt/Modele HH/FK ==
  note: gkm
  note: (Vm-Vk0)
  FKIn : Inport  Port=1  LatchInput=off
  (Vm-Vk0) : Fcn  Expr=(u-Vk)
  Product : Product
  n(Vm) : Subsystem
  n^4 : Fcn  Expr=gk*(u^4)
  FKout : Outport  InitialOutput=0
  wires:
  n(Vm)/1(n) -> n^4/1
  (Vm-Vk0)/1 -> Product/2
  Product/1 -> FKout/1
  n^4/1 -> Product/1
  FKIn/1 -> n(Vm)/1(Vm), (Vm-Vk0)/1

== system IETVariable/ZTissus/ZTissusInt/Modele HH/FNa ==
  note: gNa*m^3
  note: m
  note: h
  note: gNam
  note: (Vm-VNa0)
  FNaIn : Inport  Port=1  LatchInput=off
  (Vm-VNa0) : Fcn  Expr=(u-Vna)
  Product : Product
  Product1 : Product
  gna*m^3 : Fcn  Expr=gna*u^3
  h(Vm) : Subsystem
  m(Vm) : Subsystem
  FNaOut : Outport  InitialOutput=0
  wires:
  (Vm-VNa0)/1 -> Product1/2
  gna*m^3/1 -> Product/1
  Product1/1 -> FNaOut/1
  FNaIn/1 -> m(Vm)/1(Vm), h(Vm)/1(Vm), (Vm-VNa0)/1
  m(Vm)/1(n) -> gna*m^3/1
  h(Vm)/1(h) -> Product/2
  Product/1 -> Product1/1

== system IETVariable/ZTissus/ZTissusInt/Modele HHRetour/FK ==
  note: gkm
  note: (Vm-Vk0)
  FKIn : Inport  Port=1  LatchInput=off
  (Vm-Vk0) : Fcn  Expr=(u-Vk)
  Product : Product
  n(Vm) : Subsystem
  n^4 : Fcn  Expr=gk*(u^4)
  FKout : Outport  InitialOutput=0
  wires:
  n(Vm)/1(n) -> n^4/1
  (Vm-Vk0)/1 -> Product/2
  Product/1 -> FKout/1
  n^4/1 -> Product/1
  FKIn/1 -> n(Vm)/1(Vm), (Vm-Vk0)/1

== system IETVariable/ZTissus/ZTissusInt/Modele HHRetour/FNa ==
  note: gNa*m^3
  note: m
  note: h
  note: gNam
  note: (Vm-VNa0)
  FNaIn : Inport  Port=1  LatchInput=off
  (Vm-VNa0) : Fcn  Expr=(u-Vna)
  Product : Product
  Product1 : Product
  gna*m^3 : Fcn  Expr=gna*u^3
  h(Vm) : Subsystem
  m(Vm) : Subsystem
  FNaOut : Outport  InitialOutput=0
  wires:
  (Vm-VNa0)/1 -> Product1/2
  gna*m^3/1 -> Product/1
  Product1/1 -> FNaOut/1
  FNaIn/1 -> m(Vm)/1(Vm), h(Vm)/1(Vm), (Vm-VNa0)/1
  m(Vm)/1(n) -> gna*m^3/1
  h(Vm)/1(h) -> Product/2
  Product/1 -> Product1/1

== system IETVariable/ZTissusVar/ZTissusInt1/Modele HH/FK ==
  note: gkm
  note: (Vm-Vk0)
  FKIn : Inport  Port=1  LatchInput=off
  (Vm-Vk0) : Fcn  Expr=(u-Vk)
  Product : Product
  n(Vm) : Subsystem
  n^4 : Fcn  Expr=gk*(u^4)
  FKout : Outport  InitialOutput=0
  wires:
  n(Vm)/1(n) -> n^4/1
  (Vm-Vk0)/1 -> Product/2
  Product/1 -> FKout/1
  n^4/1 -> Product/1
  FKIn/1 -> n(Vm)/1(Vm), (Vm-Vk0)/1

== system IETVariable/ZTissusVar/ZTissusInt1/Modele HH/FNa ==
  note: gNa*m^3
  note: m
  note: h
  note: gNam
  note: (Vm-VNa0)
  FNaIn : Inport  Port=1  LatchInput=off
  (Vm-VNa0) : Fcn  Expr=(u-Vna)
  Product : Product
  Product1 : Product
  gna*m^3 : Fcn  Expr=gna*u^3
  h(Vm) : Subsystem
  m(Vm) : Subsystem
  FNaOut : Outport  InitialOutput=0
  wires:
  (Vm-VNa0)/1 -> Product1/2
  gna*m^3/1 -> Product/1
  Product1/1 -> FNaOut/1
  FNaIn/1 -> m(Vm)/1(Vm), h(Vm)/1(Vm), (Vm-VNa0)/1
  m(Vm)/1(n) -> gna*m^3/1
  h(Vm)/1(h) -> Product/2
  Product/1 -> Product1/1

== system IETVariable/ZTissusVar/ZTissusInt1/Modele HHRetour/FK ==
  note: gkm
  note: (Vm-Vk0)
  FKIn : Inport  Port=1  LatchInput=off
  (Vm-Vk0) : Fcn  Expr=(u-Vk)
  Product : Product
  n(Vm) : Subsystem
  n^4 : Fcn  Expr=gk*(u^4)
  FKout : Outport  InitialOutput=0
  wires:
  n(Vm)/1(n) -> n^4/1
  (Vm-Vk0)/1 -> Product/2
  Product/1 -> FKout/1
  n^4/1 -> Product/1
  FKIn/1 -> n(Vm)/1(Vm), (Vm-Vk0)/1

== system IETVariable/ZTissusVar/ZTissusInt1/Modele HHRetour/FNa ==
  note: gNa*m^3
  note: m
  note: h
  note: gNam
  note: (Vm-VNa0)
  FNaIn : Inport  Port=1  LatchInput=off
  (Vm-VNa0) : Fcn  Expr=(u-Vna)
  Product : Product
  Product1 : Product
  gna*m^3 : Fcn  Expr=gna*u^3
  h(Vm) : Subsystem
  m(Vm) : Subsystem
  FNaOut : Outport  InitialOutput=0
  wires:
  (Vm-VNa0)/1 -> Product1/2
  gna*m^3/1 -> Product/1
  Product1/1 -> FNaOut/1
  FNaIn/1 -> m(Vm)/1(Vm), h(Vm)/1(Vm), (Vm-VNa0)/1
  m(Vm)/1(n) -> gna*m^3/1
  h(Vm)/1(h) -> Product/2
  Product/1 -> Product1/1

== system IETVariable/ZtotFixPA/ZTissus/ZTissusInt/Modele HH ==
  HHin : Inport  Port=1  LatchInput=off
  VRefIn : Inport  Port=2  LatchInput=off
  FK : Subsystem
  FL : Fcn  Expr=gl*(u-Vl)
  FNa : Subsystem
  Gain : Gain  Gain=(1-b)/C
  Gain1 : Gain  Gain=1/(Sm*(1-b))
  Gain2 : Gain  Gain=1+mK*(b/(1-b))
  Gain3 : Gain  Gain=1+mL*(b/(1-b))
  Gain4 : Gain  Gain=1+mNa*(b/(1-b))
  Integrator : Integrator  InitialCondition=Vr
  Sum : Sum  Inputs=|---+
  Sum1 : Sum  Inputs=|++
  HHout : Outport
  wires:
  Sum/1 -> Gain/1
  Gain/1 -> Integrator/1
  FK/1(FKout) -> Gain4/1
  FNa/1(FNaOut) -> Gain2/1
  FL/1 -> Gain3/1
  HHin/1 -> Gain1/1
  Integrator/1 -> Sum1/1
  Sum1/1 -> HHout/1, FNa/1(FNaIn), FL/1, FK/1(FKIn)
  VRefIn/1 -> Sum1/2
  Gain1/1 -> Sum/4
  Gain4/1 -> Sum/1
  Gain2/1 -> Sum/2
  Gain3/1 -> Sum/3

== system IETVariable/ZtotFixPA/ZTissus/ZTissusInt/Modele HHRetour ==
  HHin : Inport  Port=1  LatchInput=off
  VRefIn : Inport  Port=2  LatchInput=off
  FK : Subsystem
  FL : Fcn  Expr=gl*(u-Vl)
  FNa : Subsystem
  Gain : Gain  Gain=(1-b)/C
  Gain1 : Gain  Gain=1/(Sm*(1-b)*Fact)
  Gain2 : Gain  Gain=1+mK*(b/(1-b))
  Gain3 : Gain  Gain=1+mL*(b/(1-b))
  Gain4 : Gain  Gain=1+mNa*(b/(1-b))
  Integrator : Integrator  InitialCondition=Vr
  Sum : Sum  Inputs=|---+
  Sum1 : Sum  Inputs=|++
  Sum2 : Sum  Inputs=|+-
  HHout : Outport
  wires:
  Sum/1 -> Gain/1
  Gain/1 -> Integrator/1
  FK/1(FKout) -> Gain4/1
  FNa/1(FNaOut) -> Gain2/1
  FL/1 -> Gain3/1
  HHin/1 -> Gain1/1
  Integrator/1 -> Sum1/1
  Sum1/1 -> FNa/1(FNaIn), FL/1, FK/1(FKIn), Sum2/1
  VRefIn/1 -> Sum1/2, Sum2/2
  Gain1/1 -> Sum/4
  Gain4/1 -> Sum/1
  Gain2/1 -> Sum/2
  Gain3/1 -> Sum/3
  Sum2/1 -> HHout/1

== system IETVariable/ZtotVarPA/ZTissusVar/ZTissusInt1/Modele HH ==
  HHin : Inport  Port=1  LatchInput=off
  VRefIn : Inport  Port=2  LatchInput=off
  FK : Subsystem
  FL : Fcn  Expr=gl*(u-Vl)
  FNa : Subsystem
  Gain : Gain  Gain=(1-b)/C
  Gain1 : Gain  Gain=1/(Sm*(1-b))
  Gain2 : Gain  Gain=1+mK*(b/(1-b))
  Gain3 : Gain  Gain=1+mL*(b/(1-b))
  Gain4 : Gain  Gain=1+mNa*(b/(1-b))
  Integrator : Integrator  InitialCondition=Vr
  Sum : Sum  Inputs=|---+
  Sum1 : Sum  Inputs=|++
  HHout : Outport
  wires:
  Sum/1 -> Gain/1
  Gain/1 -> Integrator/1
  FK/1(FKout) -> Gain4/1
  FNa/1(FNaOut) -> Gain2/1
  FL/1 -> Gain3/1
  HHin/1 -> Gain1/1
  Integrator/1 -> Sum1/1
  Sum1/1 -> HHout/1, FNa/1(FNaIn), FL/1, FK/1(FKIn)
  VRefIn/1 -> Sum1/2
  Gain1/1 -> Sum/4
  Gain4/1 -> Sum/1
  Gain2/1 -> Sum/2
  Gain3/1 -> Sum/3

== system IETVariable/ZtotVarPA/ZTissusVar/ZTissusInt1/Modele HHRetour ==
  HHin : Inport  Port=1  LatchInput=off
  VRefIn : Inport  Port=2  LatchInput=off
  FK : Subsystem
  FL : Fcn  Expr=gl*(u-Vl)
  FNa : Subsystem
  Gain : Gain  Gain=(1-b)/C
  Gain1 : Gain  Gain=1/(Sm*(1-b)*Fact)
  Gain2 : Gain  Gain=1+mK*(b/(1-b))
  Gain3 : Gain  Gain=1+mL*(b/(1-b))
  Gain4 : Gain  Gain=1+mNa*(b/(1-b))
  Integrator : Integrator  InitialCondition=Vr
  Sum : Sum  Inputs=|---+
  Sum1 : Sum  Inputs=|++
  Sum2 : Sum  Inputs=|+-
  HHout : Outport
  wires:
  Sum/1 -> Gain/1
  Gain/1 -> Integrator/1
  FK/1(FKout) -> Gain4/1
  FNa/1(FNaOut) -> Gain2/1
  FL/1 -> Gain3/1
  HHin/1 -> Gain1/1
  Integrator/1 -> Sum1/1
  Sum1/1 -> FNa/1(FNaIn), FL/1, FK/1(FKIn), Sum2/1
  VRefIn/1 -> Sum1/2, Sum2/2
  Gain1/1 -> Sum/4
  Gain4/1 -> Sum/1
  Gain2/1 -> Sum/2
  Gain3/1 -> Sum/3
  Sum2/1 -> HHout/1

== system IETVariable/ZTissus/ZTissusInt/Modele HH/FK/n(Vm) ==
  note: V
  note: alpha_*(1-n)
  note: beta_n*n
  note: n
  note: n
  Vm : Inport  Port=1  LatchInput=off
  (1-n) : Fcn  Expr=1-u
  Integrator1 : Integrator  InitialCondition=n0
  Product : Product
  Product1 : Product
  Sum1 : Sum  Inputs=+-
  V : Fcn  Expr=u-Vr
  alpha_n : Fcn  Expr=(0.01*(10-u))/(exp((10-u)/10)-1)
  beta_n : Fcn  Expr=0.125*exp(-u/80)
  n : Outport  InitialOutput=0
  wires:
  V/1 -> alpha_n/1, beta_n/1
  alpha_n/1 -> Product/2
  (1-n)/1 -> Product/1
  beta_n/1 -> Product1/1
  Product/1 -> Sum1/1
  Product1/1 -> Sum1/2
  Sum1/1 -> Integrator1/1
  Integrator1/1 -> (1-n)/1, Product1/2, n/1
  Vm/1 -> V/1

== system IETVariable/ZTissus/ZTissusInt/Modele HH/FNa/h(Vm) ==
  note: h
  note: h
  note: beta_h*h
  note: alpha_h*(1-h)
  note: V
  Vm : Inport  Port=1  LatchInput=off
  (1-h) : Fcn  Expr=1-u
  Integrator1 : Integrator  InitialCondition=h0
  Product : Product
  Product1 : Product
  Sum1 : Sum  Inputs=+-
  V : Fcn  Expr=u-Vr
  alpha_h : Fcn  Expr=0.07*exp(-u/20)
  beta_h : Fcn  Expr=1/(exp((30-u)/10)+1)
  h : Outport  InitialOutput=0
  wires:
  Vm/1 -> V/1
  Integrator1/1 -> h/1, Product1/2, (1-h)/1
  Sum1/1 -> Integrator1/1
  Product1/1 -> Sum1/2
  Product/1 -> Sum1/1
  beta_h/1 -> Product1/1
  (1-h)/1 -> Product/1
  alpha_h/1 -> Product/2
  V/1 -> beta_h/1, alpha_h/1

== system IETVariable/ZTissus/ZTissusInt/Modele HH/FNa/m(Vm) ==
  note: m
  note: m
  note: beta_m*m
  note: alpha_m*(1-m)
  note: V
  Vm : Inport  Port=1  LatchInput=off
  (1-m) : Fcn  Expr=1-u
  Integrator1 : Integrator  InitialCondition=m0
  Product : Product
  Product1 : Product
  Sum1 : Sum  Inputs=+-
  V : Fcn  Expr=u-Vr
  alpha_m : Fcn  Expr=(0.1*(25-u))/(exp((25-u)/10)-1)
  beta_m : Fcn  Expr=4*exp(-u/18)
  n : Outport  InitialOutput=0
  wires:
  Vm/1 -> V/1
  Integrator1/1 -> n/1, Product1/2, (1-m)/1
  Sum1/1 -> Integrator1/1
  Product1/1 -> Sum1/2
  Product/1 -> Sum1/1
  beta_m/1 -> Product1/1
  (1-m)/1 -> Product/1
  alpha_m/1 -> Product/2
  V/1 -> beta_m/1, alpha_m/1

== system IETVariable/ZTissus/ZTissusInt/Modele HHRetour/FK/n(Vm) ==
  note: V
  note: alpha_*(1-n)
  note: beta_n*n
  note: n
  note: n
  Vm : Inport  Port=1  LatchInput=off
  (1-n) : Fcn  Expr=1-u
  Integrator1 : Integrator  InitialCondition=n0
  Product : Product
  Product1 : Product
  Sum1 : Sum  Inputs=+-
  V : Fcn  Expr=u-Vr
  alpha_n : Fcn  Expr=(0.01*(10-u))/(exp((10-u)/10)-1)
  beta_n : Fcn  Expr=0.125*exp(-u/80)
  n : Outport  InitialOutput=0
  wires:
  V/1 -> alpha_n/1, beta_n/1
  alpha_n/1 -> Product/2
  (1-n)/1 -> Product/1
  beta_n/1 -> Product1/1
  Product/1 -> Sum1/1
  Product1/1 -> Sum1/2
  Sum1/1 -> Integrator1/1
  Integrator1/1 -> (1-n)/1, Product1/2, n/1
  Vm/1 -> V/1

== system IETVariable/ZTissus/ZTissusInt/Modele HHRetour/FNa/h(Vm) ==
  note: h
  note: h
  note: beta_h*h
  note: alpha_h*(1-h)
  note: V
  Vm : Inport  Port=1  LatchInput=off
  (1-h) : Fcn  Expr=1-u
  Integrator1 : Integrator  InitialCondition=h0
  Product : Product
  Product1 : Product
  Sum1 : Sum  Inputs=+-
  V : Fcn  Expr=u-Vr
  alpha_h : Fcn  Expr=0.07*exp(-u/20)
  beta_h : Fcn  Expr=1/(exp((30-u)/10)+1)
  h : Outport  InitialOutput=0
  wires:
  Vm/1 -> V/1
  Integrator1/1 -> h/1, Product1/2, (1-h)/1
  Sum1/1 -> Integrator1/1
  Product1/1 -> Sum1/2
  Product/1 -> Sum1/1
  beta_h/1 -> Product1/1
  (1-h)/1 -> Product/1
  alpha_h/1 -> Product/2
  V/1 -> beta_h/1, alpha_h/1

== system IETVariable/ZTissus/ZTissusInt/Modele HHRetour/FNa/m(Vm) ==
  note: m
  note: m
  note: beta_m*m
  note: alpha_m*(1-m)
  note: V
  Vm : Inport  Port=1  LatchInput=off
  (1-m) : Fcn  Expr=1-u
  Integrator1 : Integrator  InitialCondition=m0
  Product : Product
  Product1 : Product
  Sum1 : Sum  Inputs=+-
  V : Fcn  Expr=u-Vr
  alpha_m : Fcn  Expr=(0.1*(25-u))/(exp((25-u)/10)-1)
  beta_m : Fcn  Expr=4*exp(-u/18)
  n : Outport  InitialOutput=0
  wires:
  Vm/1 -> V/1
  Integrator1/1 -> n/1, Product1/2, (1-m)/1
  Sum1/1 -> Integrator1/1
  Product1/1 -> Sum1/2
  Product/1 -> Sum1/1
  beta_m/1 -> Product1/1
  (1-m)/1 -> Product/1
  alpha_m/1 -> Product/2
  V/1 -> beta_m/1, alpha_m/1

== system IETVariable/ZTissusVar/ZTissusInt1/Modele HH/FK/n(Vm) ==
  note: V
  note: alpha_*(1-n)
  note: beta_n*n
  note: n
  note: n
  Vm : Inport  Port=1  LatchInput=off
  (1-n) : Fcn  Expr=1-u
  Integrator1 : Integrator  InitialCondition=n0
  Product : Product
  Product1 : Product
  Sum1 : Sum  Inputs=+-
  V : Fcn  Expr=u-Vr
  alpha_n : Fcn  Expr=(0.01*(10-u))/(exp((10-u)/10)-1)
  beta_n : Fcn  Expr=0.125*exp(-u/80)
  n : Outport  InitialOutput=0
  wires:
  V/1 -> alpha_n/1, beta_n/1
  alpha_n/1 -> Product/2
  (1-n)/1 -> Product/1
  beta_n/1 -> Product1/1
  Product/1 -> Sum1/1
  Product1/1 -> Sum1/2
  Sum1/1 -> Integrator1/1
  Integrator1/1 -> (1-n)/1, Product1/2, n/1
  Vm/1 -> V/1

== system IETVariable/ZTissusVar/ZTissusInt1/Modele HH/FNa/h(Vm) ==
  note: h
  note: h
  note: beta_h*h
  note: alpha_h*(1-h)
  note: V
  Vm : Inport  Port=1  LatchInput=off
  (1-h) : Fcn  Expr=1-u
  Integrator1 : Integrator  InitialCondition=h0
  Product : Product
  Product1 : Product
  Sum1 : Sum  Inputs=+-
  V : Fcn  Expr=u-Vr
  alpha_h : Fcn  Expr=0.07*exp(-u/20)
  beta_h : Fcn  Expr=1/(exp((30-u)/10)+1)
  h : Outport  InitialOutput=0
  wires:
  Vm/1 -> V/1
  Integrator1/1 -> h/1, Product1/2, (1-h)/1
  Sum1/1 -> Integrator1/1
  Product1/1 -> Sum1/2
  Product/1 -> Sum1/1
  beta_h/1 -> Product1/1
  (1-h)/1 -> Product/1
  alpha_h/1 -> Product/2
  V/1 -> beta_h/1, alpha_h/1

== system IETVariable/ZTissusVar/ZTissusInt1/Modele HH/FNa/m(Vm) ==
  note: m
  note: m
  note: beta_m*m
  note: alpha_m*(1-m)
  note: V
  Vm : Inport  Port=1  LatchInput=off
  (1-m) : Fcn  Expr=1-u
  Integrator1 : Integrator  InitialCondition=m0
  Product : Product
  Product1 : Product
  Sum1 : Sum  Inputs=+-
  V : Fcn  Expr=u-Vr
  alpha_m : Fcn  Expr=(0.1*(25-u))/(exp((25-u)/10)-1)
  beta_m : Fcn  Expr=4*exp(-u/18)
  n : Outport  InitialOutput=0
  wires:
  Vm/1 -> V/1
  Integrator1/1 -> n/1, Product1/2, (1-m)/1
  Sum1/1 -> Integrator1/1
  Product1/1 -> Sum1/2
  Product/1 -> Sum1/1
  beta_m/1 -> Product1/1
  (1-m)/1 -> Product/1
  alpha_m/1 -> Product/2
  V/1 -> beta_m/1, alpha_m/1

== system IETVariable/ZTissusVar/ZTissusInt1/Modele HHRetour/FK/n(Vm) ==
  note: V
  note: alpha_*(1-n)
  note: beta_n*n
  note: n
  note: n
  Vm : Inport  Port=1  LatchInput=off
  (1-n) : Fcn  Expr=1-u
  Integrator1 : Integrator  InitialCondition=n0
  Product : Product
  Product1 : Product
  Sum1 : Sum  Inputs=+-
  V : Fcn  Expr=u-Vr
  alpha_n : Fcn  Expr=(0.01*(10-u))/(exp((10-u)/10)-1)
  beta_n : Fcn  Expr=0.125*exp(-u/80)
  n : Outport  InitialOutput=0
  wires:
  V/1 -> alpha_n/1, beta_n/1
  alpha_n/1 -> Product/2
  (1-n)/1 -> Product/1
  beta_n/1 -> Product1/1
  Product/1 -> Sum1/1
  Product1/1 -> Sum1/2
  Sum1/1 -> Integrator1/1
  Integrator1/1 -> (1-n)/1, Product1/2, n/1
  Vm/1 -> V/1

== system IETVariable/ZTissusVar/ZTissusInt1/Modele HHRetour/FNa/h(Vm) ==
  note: h
  note: h
  note: beta_h*h
  note: alpha_h*(1-h)
  note: V
  Vm : Inport  Port=1  LatchInput=off
  (1-h) : Fcn  Expr=1-u
  Integrator1 : Integrator  InitialCondition=h0
  Product : Product
  Product1 : Product
  Sum1 : Sum  Inputs=+-
  V : Fcn  Expr=u-Vr
  alpha_h : Fcn  Expr=0.07*exp(-u/20)
  beta_h : Fcn  Expr=1/(exp((30-u)/10)+1)
  h : Outport  InitialOutput=0
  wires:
  Vm/1 -> V/1
  Integrator1/1 -> h/1, Product1/2, (1-h)/1
  Sum1/1 -> Integrator1/1
  Product1/1 -> Sum1/2
  Product/1 -> Sum1/1
  beta_h/1 -> Product1/1
  (1-h)/1 -> Product/1
  alpha_h/1 -> Product/2
  V/1 -> beta_h/1, alpha_h/1

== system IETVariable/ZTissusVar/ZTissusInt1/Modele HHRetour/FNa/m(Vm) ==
  note: m
  note: m
  note: beta_m*m
  note: alpha_m*(1-m)
  note: V
  Vm : Inport  Port=1  LatchInput=off
  (1-m) : Fcn  Expr=1-u
  Integrator1 : Integrator  InitialCondition=m0
  Product : Product
  Product1 : Product
  Sum1 : Sum  Inputs=+-
  V : Fcn  Expr=u-Vr
  alpha_m : Fcn  Expr=(0.1*(25-u))/(exp((25-u)/10)-1)
  beta_m : Fcn  Expr=4*exp(-u/18)
  n : Outport  InitialOutput=0
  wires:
  Vm/1 -> V/1
  Integrator1/1 -> n/1, Product1/2, (1-m)/1
  Sum1/1 -> Integrator1/1
  Product1/1 -> Sum1/2
  Product/1 -> Sum1/1
  beta_m/1 -> Product1/1
  (1-m)/1 -> Product/1
  alpha_m/1 -> Product/2
  V/1 -> beta_m/1, alpha_m/1

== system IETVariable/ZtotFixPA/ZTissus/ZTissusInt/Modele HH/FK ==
  note: gkm
  note: (Vm-Vk0)
  FKIn : Inport  Port=1  LatchInput=off
  (Vm-Vk0) : Fcn  Expr=(u-Vk)
  Product : Product
  n(Vm) : Subsystem
  n^4 : Fcn  Expr=gk*(u^4)
  FKout : Outport  InitialOutput=0
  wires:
  n(Vm)/1(n) -> n^4/1
  (Vm-Vk0)/1 -> Product/2
  Product/1 -> FKout/1
  n^4/1 -> Product/1
  FKIn/1 -> n(Vm)/1(Vm), (Vm-Vk0)/1

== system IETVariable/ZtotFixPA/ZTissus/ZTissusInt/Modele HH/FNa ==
  note: gNa*m^3
  note: m
  note: h
  note: gNam
  note: (Vm-VNa0)
  FNaIn : Inport  Port=1  LatchInput=off
  (Vm-VNa0) : Fcn  Expr=(u-Vna)
  Product : Product
  Product1 : Product
  gna*m^3 : Fcn  Expr=gna*u^3
  h(Vm) : Subsystem
  m(Vm) : Subsystem
  FNaOut : Outport  InitialOutput=0
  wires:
  (Vm-VNa0)/1 -> Product1/2
  gna*m^3/1 -> Product/1
  Product1/1 -> FNaOut/1
  FNaIn/1 -> m(Vm)/1(Vm), h(Vm)/1(Vm), (Vm-VNa0)/1
  m(Vm)/1(n) -> gna*m^3/1
  h(Vm)/1(h) -> Product/2
  Product/1 -> Product1/1

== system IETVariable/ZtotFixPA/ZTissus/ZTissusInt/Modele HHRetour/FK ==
  note: gkm
  note: (Vm-Vk0)
  FKIn : Inport  Port=1  LatchInput=off
  (Vm-Vk0) : Fcn  Expr=(u-Vk)
  Product : Product
  n(Vm) : Subsystem
  n^4 : Fcn  Expr=gk*(u^4)
  FKout : Outport  InitialOutput=0
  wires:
  n(Vm)/1(n) -> n^4/1
  (Vm-Vk0)/1 -> Product/2
  Product/1 -> FKout/1
  n^4/1 -> Product/1
  FKIn/1 -> n(Vm)/1(Vm), (Vm-Vk0)/1

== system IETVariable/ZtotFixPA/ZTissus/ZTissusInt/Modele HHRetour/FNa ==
  note: gNa*m^3
  note: m
  note: h
  note: gNam
  note: (Vm-VNa0)
  FNaIn : Inport  Port=1  LatchInput=off
  (Vm-VNa0) : Fcn  Expr=(u-Vna)
  Product : Product
  Product1 : Product
  gna*m^3 : Fcn  Expr=gna*u^3
  h(Vm) : Subsystem
  m(Vm) : Subsystem
  FNaOut : Outport  InitialOutput=0
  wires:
  (Vm-VNa0)/1 -> Product1/2
  gna*m^3/1 -> Product/1
  Product1/1 -> FNaOut/1
  FNaIn/1 -> m(Vm)/1(Vm), h(Vm)/1(Vm), (Vm-VNa0)/1
  m(Vm)/1(n) -> gna*m^3/1
  h(Vm)/1(h) -> Product/2
  Product/1 -> Product1/1

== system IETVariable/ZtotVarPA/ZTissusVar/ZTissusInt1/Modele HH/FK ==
  note: gkm
  note: (Vm-Vk0)
  FKIn : Inport  Port=1  LatchInput=off
  (Vm-Vk0) : Fcn  Expr=(u-Vk)
  Product : Product
  n(Vm) : Subsystem
  n^4 : Fcn  Expr=gk*(u^4)
  FKout : Outport  InitialOutput=0
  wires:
  n(Vm)/1(n) -> n^4/1
  (Vm-Vk0)/1 -> Product/2
  Product/1 -> FKout/1
  n^4/1 -> Product/1
  FKIn/1 -> n(Vm)/1(Vm), (Vm-Vk0)/1

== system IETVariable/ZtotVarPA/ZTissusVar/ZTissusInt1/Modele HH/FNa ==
  note: gNa*m^3
  note: m
  note: h
  note: gNam
  note: (Vm-VNa0)
  FNaIn : Inport  Port=1  LatchInput=off
  (Vm-VNa0) : Fcn  Expr=(u-Vna)
  Product : Product
  Product1 : Product
  gna*m^3 : Fcn  Expr=gna*u^3
  h(Vm) : Subsystem
  m(Vm) : Subsystem
  FNaOut : Outport  InitialOutput=0
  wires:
  (Vm-VNa0)/1 -> Product1/2
  gna*m^3/1 -> Product/1
  Product1/1 -> FNaOut/1
  FNaIn/1 -> m(Vm)/1(Vm), h(Vm)/1(Vm), (Vm-VNa0)/1
  m(Vm)/1(n) -> gna*m^3/1
  h(Vm)/1(h) -> Product/2
  Product/1 -> Product1/1

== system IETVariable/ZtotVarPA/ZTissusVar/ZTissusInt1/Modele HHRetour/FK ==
  note: gkm
  note: (Vm-Vk0)
  FKIn : Inport  Port=1  LatchInput=off
  (Vm-Vk0) : Fcn  Expr=(u-Vk)
  Product : Product
  n(Vm) : Subsystem
  n^4 : Fcn  Expr=gk*(u^4)
  FKout : Outport  InitialOutput=0
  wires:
  n(Vm)/1(n) -> n^4/1
  (Vm-Vk0)/1 -> Product/2
  Product/1 -> FKout/1
  n^4/1 -> Product/1
  FKIn/1 -> n(Vm)/1(Vm), (Vm-Vk0)/1

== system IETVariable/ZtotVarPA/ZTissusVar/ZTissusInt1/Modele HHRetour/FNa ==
  note: gNa*m^3
  note: m
  note: h
  note: gNam
  note: (Vm-VNa0)
  FNaIn : Inport  Port=1  LatchInput=off
  (Vm-VNa0) : Fcn  Expr=(u-Vna)
  Product : Product
  Product1 : Product
  gna*m^3 : Fcn  Expr=gna*u^3
  h(Vm) : Subsystem
  m(Vm) : Subsystem
  FNaOut : Outport  InitialOutput=0
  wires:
  (Vm-VNa0)/1 -> Product1/2
  gna*m^3/1 -> Product/1
  Product1/1 -> FNaOut/1
  FNaIn/1 -> m(Vm)/1(Vm), h(Vm)/1(Vm), (Vm-VNa0)/1
  m(Vm)/1(n) -> gna*m^3/1
  h(Vm)/1(h) -> Product/2
  Product/1 -> Product1/1

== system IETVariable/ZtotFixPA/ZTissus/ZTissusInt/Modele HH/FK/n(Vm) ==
  note: V
  note: alpha_*(1-n)
  note: beta_n*n
  note: n
  note: n
  Vm : Inport  Port=1  LatchInput=off
  (1-n) : Fcn  Expr=1-u
  Integrator1 : Integrator  InitialCondition=n0
  Product : Product
  Product1 : Product
  Sum1 : Sum  Inputs=+-
  V : Fcn  Expr=u-Vr
  alpha_n : Fcn  Expr=(0.01*(10-u))/(exp((10-u)/10)-1)
  beta_n : Fcn  Expr=0.125*exp(-u/80)
  n : Outport  InitialOutput=0
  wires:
  V/1 -> alpha_n/1, beta_n/1
  alpha_n/1 -> Product/2
  (1-n)/1 -> Product/1
  beta_n/1 -> Product1/1
  Product/1 -> Sum1/1
  Product1/1 -> Sum1/2
  Sum1/1 -> Integrator1/1
  Integrator1/1 -> (1-n)/1, Product1/2, n/1
  Vm/1 -> V/1

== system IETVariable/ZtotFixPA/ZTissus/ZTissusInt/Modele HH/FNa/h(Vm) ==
  note: h
  note: h
  note: beta_h*h
  note: alpha_h*(1-h)
  note: V
  Vm : Inport  Port=1  LatchInput=off
  (1-h) : Fcn  Expr=1-u
  Integrator1 : Integrator  InitialCondition=h0
  Product : Product
  Product1 : Product
  Sum1 : Sum  Inputs=+-
  V : Fcn  Expr=u-Vr
  alpha_h : Fcn  Expr=0.07*exp(-u/20)
  beta_h : Fcn  Expr=1/(exp((30-u)/10)+1)
  h : Outport  InitialOutput=0
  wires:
  Vm/1 -> V/1
  Integrator1/1 -> h/1, Product1/2, (1-h)/1
  Sum1/1 -> Integrator1/1
  Product1/1 -> Sum1/2
  Product/1 -> Sum1/1
  beta_h/1 -> Product1/1
  (1-h)/1 -> Product/1
  alpha_h/1 -> Product/2
  V/1 -> beta_h/1, alpha_h/1

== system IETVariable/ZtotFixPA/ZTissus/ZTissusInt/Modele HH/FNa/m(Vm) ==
  note: m
  note: m
  note: beta_m*m
  note: alpha_m*(1-m)
  note: V
  Vm : Inport  Port=1  LatchInput=off
  (1-m) : Fcn  Expr=1-u
  Integrator1 : Integrator  InitialCondition=m0
  Product : Product
  Product1 : Product
  Sum1 : Sum  Inputs=+-
  V : Fcn  Expr=u-Vr
  alpha_m : Fcn  Expr=(0.1*(25-u))/(exp((25-u)/10)-1)
  beta_m : Fcn  Expr=4*exp(-u/18)
  n : Outport  InitialOutput=0
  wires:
  Vm/1 -> V/1
  Integrator1/1 -> n/1, Product1/2, (1-m)/1
  Sum1/1 -> Integrator1/1
  Product1/1 -> Sum1/2
  Product/1 -> Sum1/1
  beta_m/1 -> Product1/1
  (1-m)/1 -> Product/1
  alpha_m/1 -> Product/2
  V/1 -> beta_m/1, alpha_m/1
